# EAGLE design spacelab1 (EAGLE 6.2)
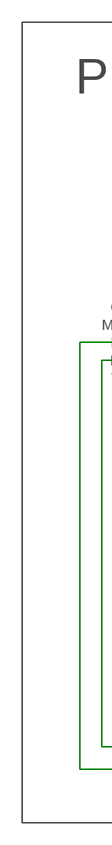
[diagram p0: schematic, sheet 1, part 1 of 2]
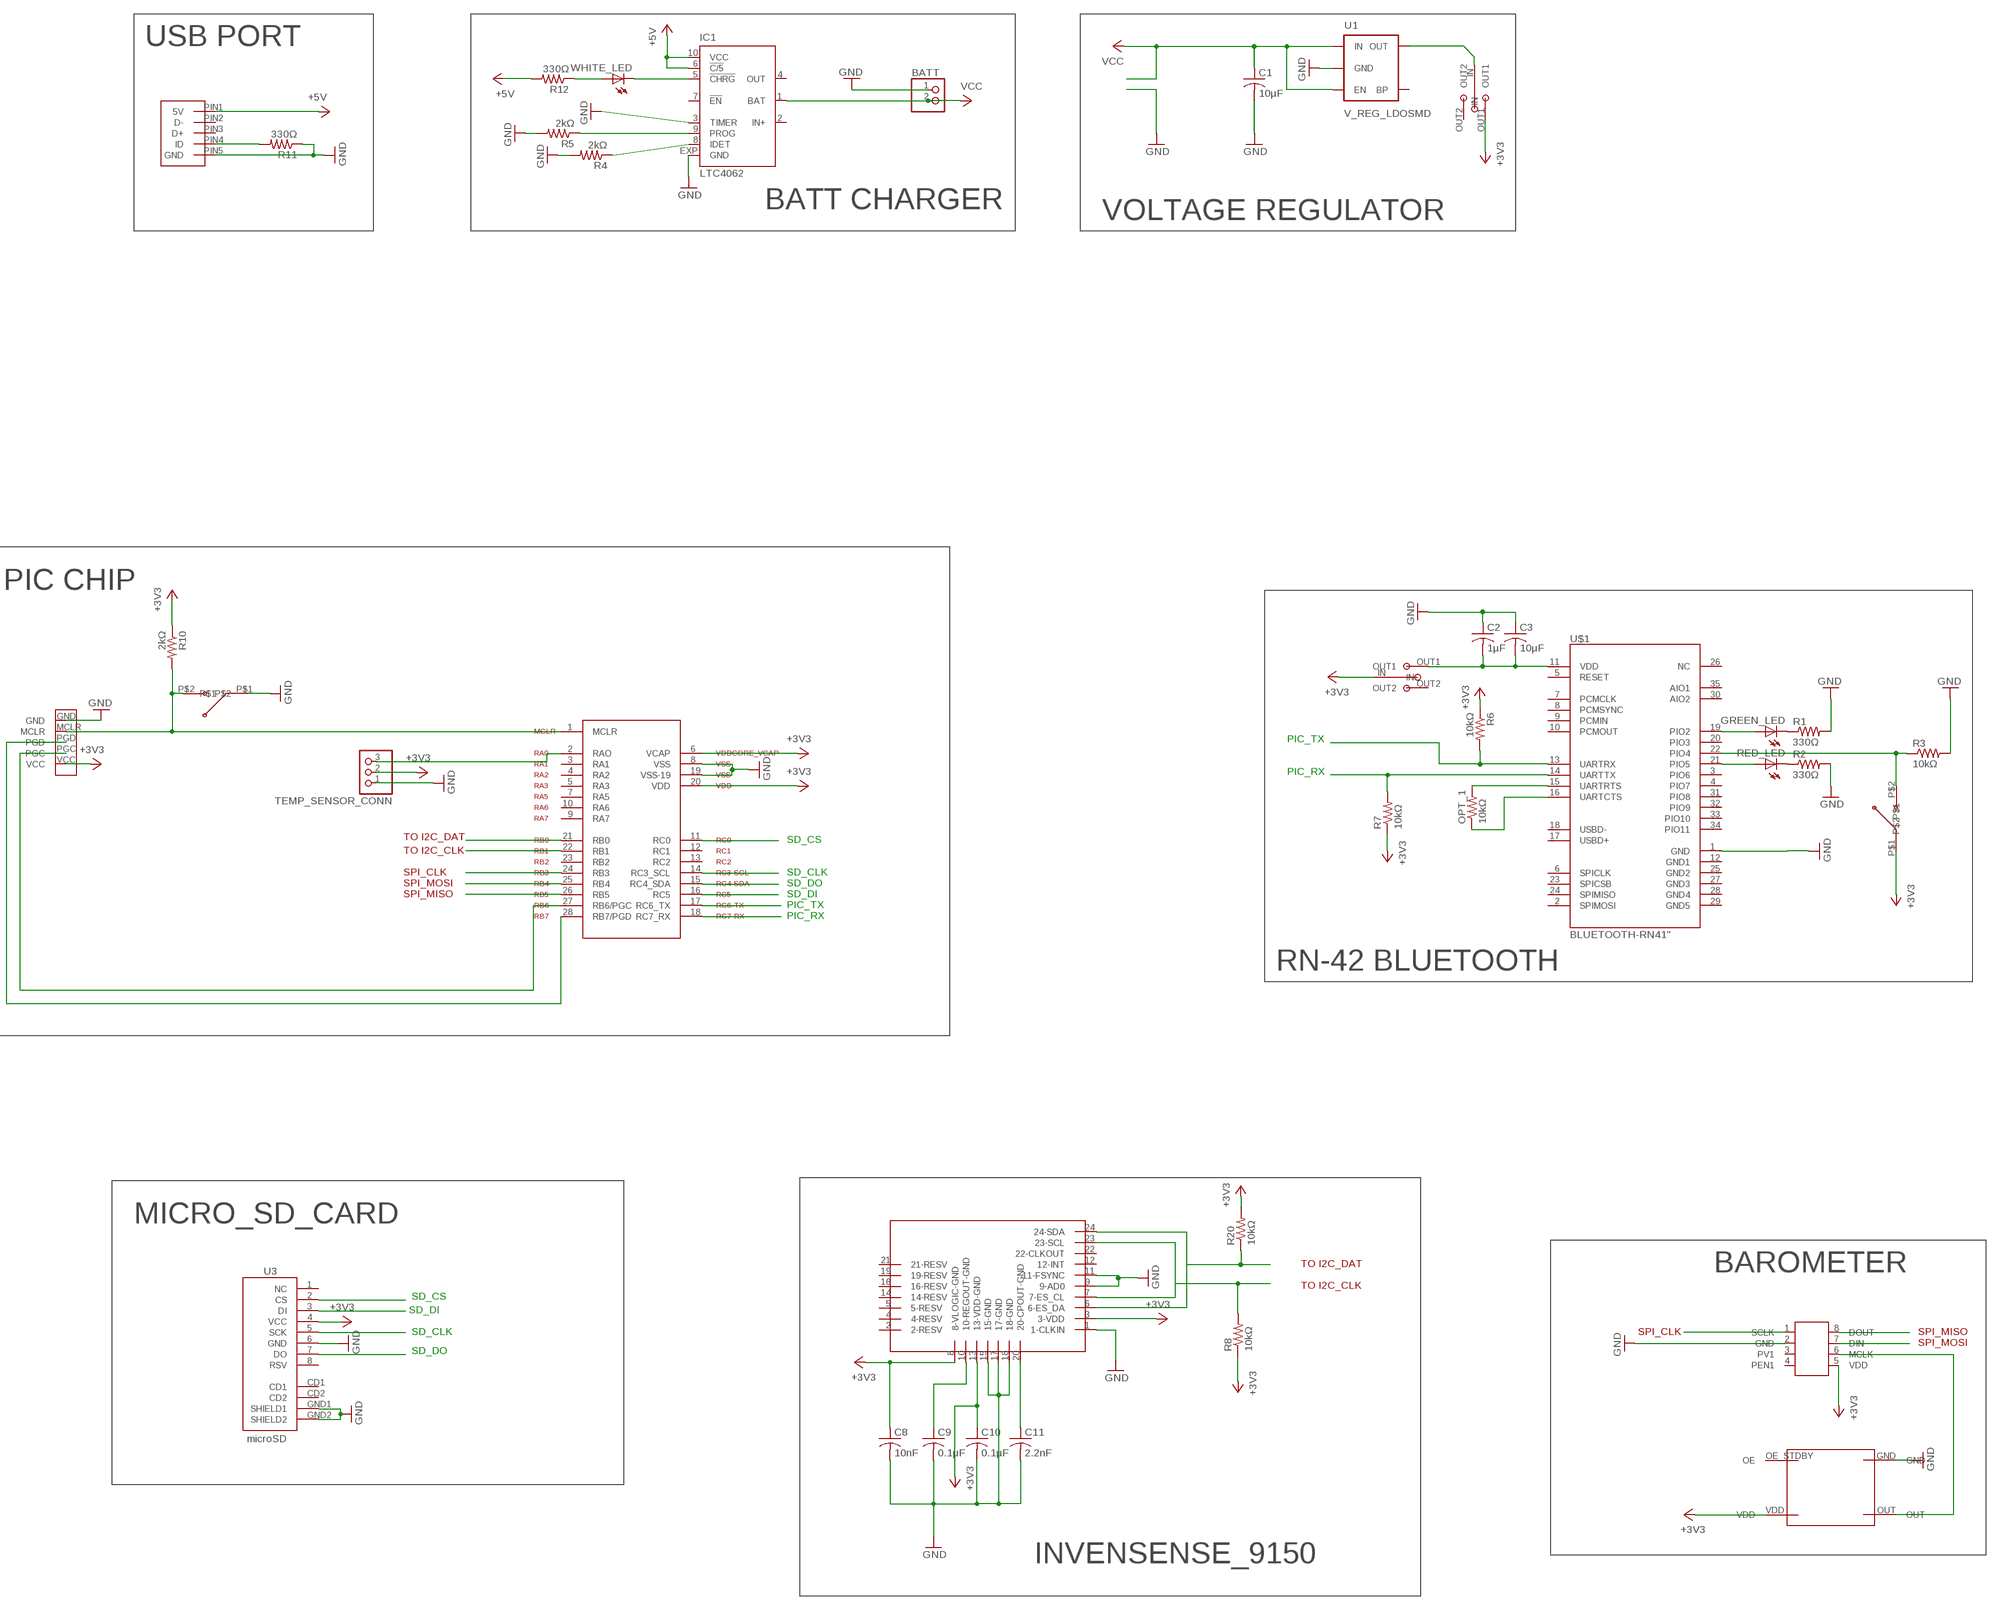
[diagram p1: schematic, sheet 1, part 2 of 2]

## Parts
BATT  PINHD-1X2  [1X02]
BT_PWR  CUS12TB_LOW_PROFILE_SWITCH  [CUS12TB_FOOTPRINT]
BT_RST  KSR211_MOM  [KSR_211_FOOTPRINT]
C1  10µF  C-USC0603  [C0603]
C2  1µF  C-USC0603  [C0603]
C3  10µF  C-USC0603  [C0603]
C8  10nF  C-USC0805  [C0805]
C9  0.1µF  C-USC0805  [C0805]
C10  0.1µF  C-USC0805  [C0805]
C11  2.2nF  C-USC0805  [C0805]
GREEN_LED  LEDCHIP-LED0805  [CHIP-LED0805]
IC1  LTC4062  [DFN10-3X3]
MAIN_PWR  CUS12TB_LOW_PROFILE_SWITCH  [CUS12TB_FOOTPRINT]
OPT_1  10kΩ  R-US_R0603  [R0603]
PIC18F26J11  PIC18F26J11  [SSOP-28]
PIC_RST  KSR211_MOM  [KSR_211_FOOTPRINT]
R1  330Ω  R-US_R0603  [R0603]
R2  330Ω  R-US_R0603  [R0603]
R3  10kΩ  R-US_R0603  [R0603]
R4  2kΩ  R-US_R0603  [R0603]
R5  2kΩ  R-US_R0603  [R0603]
R6  10kΩ  R-US_R0603  [R0603]
R7  10kΩ  R-US_R0603  [R0603]
R8  10kΩ  R-US_R0603  [R0603]
R10  2kΩ  R-US_R0603  [R0603]
R11  330Ω  R-US_R0603  [R0603]
R12  330Ω  R-US_R0603  [R0603]
R20  10kΩ  R-US_R0603  [R0603]
RED_LED  LEDCHIP-LED0805  [CHIP-LED0805]
TEMP_SENSOR_CONN  PINHD-1X3  [1X03]
U1  V_REG_LDOSMD  [SOT23-5]
U3  microSD  USD-SOCKETSMD  [MICRO-SD-SOCKET-PP]
U$1  BLUETOOTH-RN41"  [RN41]
U$2  CSX_750F_CLOCK  [CITIZEN_CSX-750_CRYSTAL_OSCILLATOR]
U$3  5-PAD_PROG_HEAD  [5-BUTTON_PAD]
U$4  INVENSENSE-MPU9150  [INVENSENSE-MPU9150]
U$5  WURTH_MICRO_USB_SMD  [MICRO_USB_SMD]
U$8  MS5540C_BAROMETER  [8_PIN_MS5540C]
WHITE_LED  LEDCHIP-LED0805  [CHIP-LED0805]

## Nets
+3V3: BT_PWR.IN BT_RST.P$1 C8.1 C10.1 MAIN_PWR.OUT1 PIC18F26J11.6(VCAP) PIC18F26J11.20(VDD) R6.1 R7.1 R8.1 R10.1 R20.2 TEMP_SENSOR_CONN.2 U3.4(VCC) U$2.VDD U$3.VCC U$4.3(3-VDD) U$4.8(8-VLOGIC-GND) U$4.13(13-VDD-GND) U$8.5(VDD)
+5V: IC1.6(!C/5) IC1.10(VCC) R12.2 U$5.PIN1(5V)
GND: BATT.1 C1.2 C2.1 C3.1 C8.2 C9.2 C10.2 C11.2 IC1.3(TIMER) IC1.EXP(GND) PIC18F26J11.8(VSS) PIC18F26J11.19(VSS-19) PIC_RST.P$1 R1.2 R2.2 R3.2 R4.2 R5.2 R11.1 TEMP_SENSOR_CONN.1 U1.2(GND) U3.6(GND) U3.GND1(SHIELD1) U3.GND2(SHIELD2) U$1.1(GND) U$2.GND U$3.GND U$4.1(1-CLKIN) U$4.9(9-AD0) U$4.11(11-FSYNC) U$4.15(15-GND) U$4.17(17-GND) U$4.18(18-GND) U$5.PIN5(GND) U$8.2(GND)
I2C_CLK: PIC18F26J11.22(RB1) R8.2 U$4.7(7-ES_CL) U$4.23(23-SCL)
I2C_DAT: PIC18F26J11.21(RB0) R20.1 U$4.6(6-ES_DA) U$4.24(24-SDA)
N$1: GREEN_LED.A U$1.19(PIO2)
N$2: RED_LED.A U$1.21(PIO5)
N$3: GREEN_LED.C R1.1
N$4: R2.1 RED_LED.C
N$5: BT_RST.P$2 R3.1 U$1.22(PIO4)
N$6: OPT_1.2 U$1.15(UARTRTS)
N$7: OPT_1.1 U$1.16(UARTCTS)
N$8: IC1.9(PROG) R5.1
N$9: IC1.8(IDET) R4.1
N$10: U$8.1(SCLK)
N$11: R11.2 U$5.PIN4(ID)
N$12: U$8.7(DIN)
N$13: PIC18F26J11.1(MCLR) PIC_RST.P$2 R10.2 U$3.MCLR
N$14: U$8.8(DOUT)
N$15: PIC18F26J11.28(RB7/PGD) U$3.PGD
N$16: PIC18F26J11.27(RB6/PGC) U$3.PGC
N$17: PIC18F26J11.2(RAO) TEMP_SENSOR_CONN.3
N$18: BT_PWR.OUT1 C2.2 C3.2 U$1.11(VDD)
N$19: U$2.OUT U$8.6(MCLK)
N$23: IC1.5(!CHRG) WHITE_LED.C
N$24: R12.1 WHITE_LED.A
N$29: MAIN_PWR.IN U1.5(OUT)
N$44: C9.1 U$4.10(10-REGOUT-GND)
N$45: C11.1 U$4.20(20-CPOUT-GND)
PIC_RX: PIC18F26J11.18(RC7_RX) R7.2 U$1.14(UARTTX)
PIC_TX: PIC18F26J11.17(RC6_TX) R6.2 U$1.13(UARTRX)
SD_CLK: PIC18F26J11.14(RC3_SCL) U3.5(SCK)
SD_CS: PIC18F26J11.11(RC0) U3.2(CS)
SD_DI: PIC18F26J11.16(RC5) U3.3(DI)
SD_DO: PIC18F26J11.15(RC4_SDA) U3.7(DO)
SPI_CLK: PIC18F26J11.24(RB3)
SPI_MISO: PIC18F26J11.26(RB5)
SPI_MOSI: PIC18F26J11.25(RB4)
VCC: BATT.2 C1.1 IC1.1(BAT) U1.1(IN) U1.3(EN)
Unconnected: BT_PWR.OUT2 IC1.2(IN+) IC1.4(OUT) IC1.7(!EN) MAIN_PWR.OUT2 PIC18F26J11.3(RA1) PIC18F26J11.4(RA2) PIC18F26J11.5(RA3) PIC18F26J11.7(RA5) PIC18F26J11.9(RA7) PIC18F26J11.10(RA6) PIC18F26J11.12(RC1) PIC18F26J11.13(RC2) PIC18F26J11.23(RB2) U1.4(BP) U3.1(NC) U3.8(RSV) U3.CD1 U3.CD2 U$1.2(SPIMOSI) U$1.3(PIO6) U$1.4(PIO7) U$1.5(RESET) U$1.6(SPICLK) U$1.7(PCMCLK) U$1.8(PCMSYNC) U$1.9(PCMIN) U$1.10(PCMOUT) U$1.12(GND1) U$1.17(USBD+) U$1.18(USBD-) U$1.20(PIO3) U$1.23(SPICSB) U$1.24(SPIMISO) U$1.25(GND2) U$1.26(NC) U$1.27(GND3) U$1.28(GND4) U$1.29(GND5) U$1.30(AIO2) U$1.31(PIO8) U$1.32(PIO9) U$1.33(PIO10) U$1.34(PIO11) U$1.35(AIO1) U$2.OE_STDBY(OE) U$4.2(2-RESV) U$4.4(4-RESV) U$4.5(5-RESV) U$4.12(12-INT) U$4.14(14-RESV) U$4.16(16-RESV) U$4.19(19-RESV) U$4.21(21-RESV) U$4.22(22-CLKOUT) U$5.PIN2(D-) U$5.PIN3(D+) U$8.3(PV1) U$8.4(PEN1)

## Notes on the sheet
- USB PORT
- BATT CHARGER
- VOLTAGE REGULATOR
- PIC CHIP
- PIC_TX
- PIC_RX
- TO I2C_DAT | SD_CS
- TO I2C_CLK
- SPI_CLK | SD_CLK
- SPI_MOSI | SD_DO
- SPI_MISO | SD_DI
- PIC_TX
- PIC_RX
- RN-42 BLUETOOTH
- MICRO_SD_CARD
- TO I2C_DAT
- BAROMETER
- TO I2C_CLK
- SD_CS
- SD_DI
- SD_CLK | SPI_CLK | SPI_MISO
- SPI_MOSI
- SD_DO
- INVENSENSE_9150

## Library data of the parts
BATT = pinhead:PINHD-1X2: PIN HEADER
BT_PWR MAIN_PWR = copal_slide_switches:CUS12TB_LOW_PROFILE_SWITCH
BT_RST PIC_RST = c_and_k_switches:KSR211_MOM
C1-C3 C8-C11 = resistor:C-US: CAPACITOR, American symbol
GREEN_LED RED_LED WHITE_LED = led:LED: LED
IC1 = linear-technology:LTC4062: Standalone Linear Li-Ion Battery Charger with Micropower Comparator Source: http://www.linear.com .. 4062fa.pdf; MPN: LTC4062EDD#PBF; OC_FARNELL: 1648037; OC_NEWARK: 58M0900
OPT_1 R1-R8 R10-R12 R20 = resistor:R-US_: RESISTOR, American symbol
PIC18F26J11 = 18F26J11:PIC18F26J11
TEMP_SENSOR_CONN = pinhead:PINHD-1X3: PIN HEADER
U1 = SparkFun-PowerIC:V_REG_LDO: Voltage Regulator LDO Standard 150mA LDO voltage regulator in SOT-23 layout. Micrel part MIC5205. BP (by-pass) pin is used to lower output noise with 470pF cap.
U3 = SparkFun:USD-SOCKET: microSD Socket Push-push type uSD socket. Schematic element and footprint production proven. Spark Fun Electronics SKU : PRT-00127. tDoc lines correctly indicate media card edge positions when inserting (unlocked, locked, depressed).
U$1 = SparkFun-RF:BLUETOOTH-RN41: Bluetooth SMD module
U$2 = citizen:CSX_750F_CLOCK
U$3 = Jeremy_Parts:5-PAD_PROG_HEAD
U$4 = vids-parts:INVENSENSE-MPU9150
U$5 = wurth_micro_usb:WURTH_MICRO_USB_SMD
U$8 = Intersema:MS5540C_BAROMETER

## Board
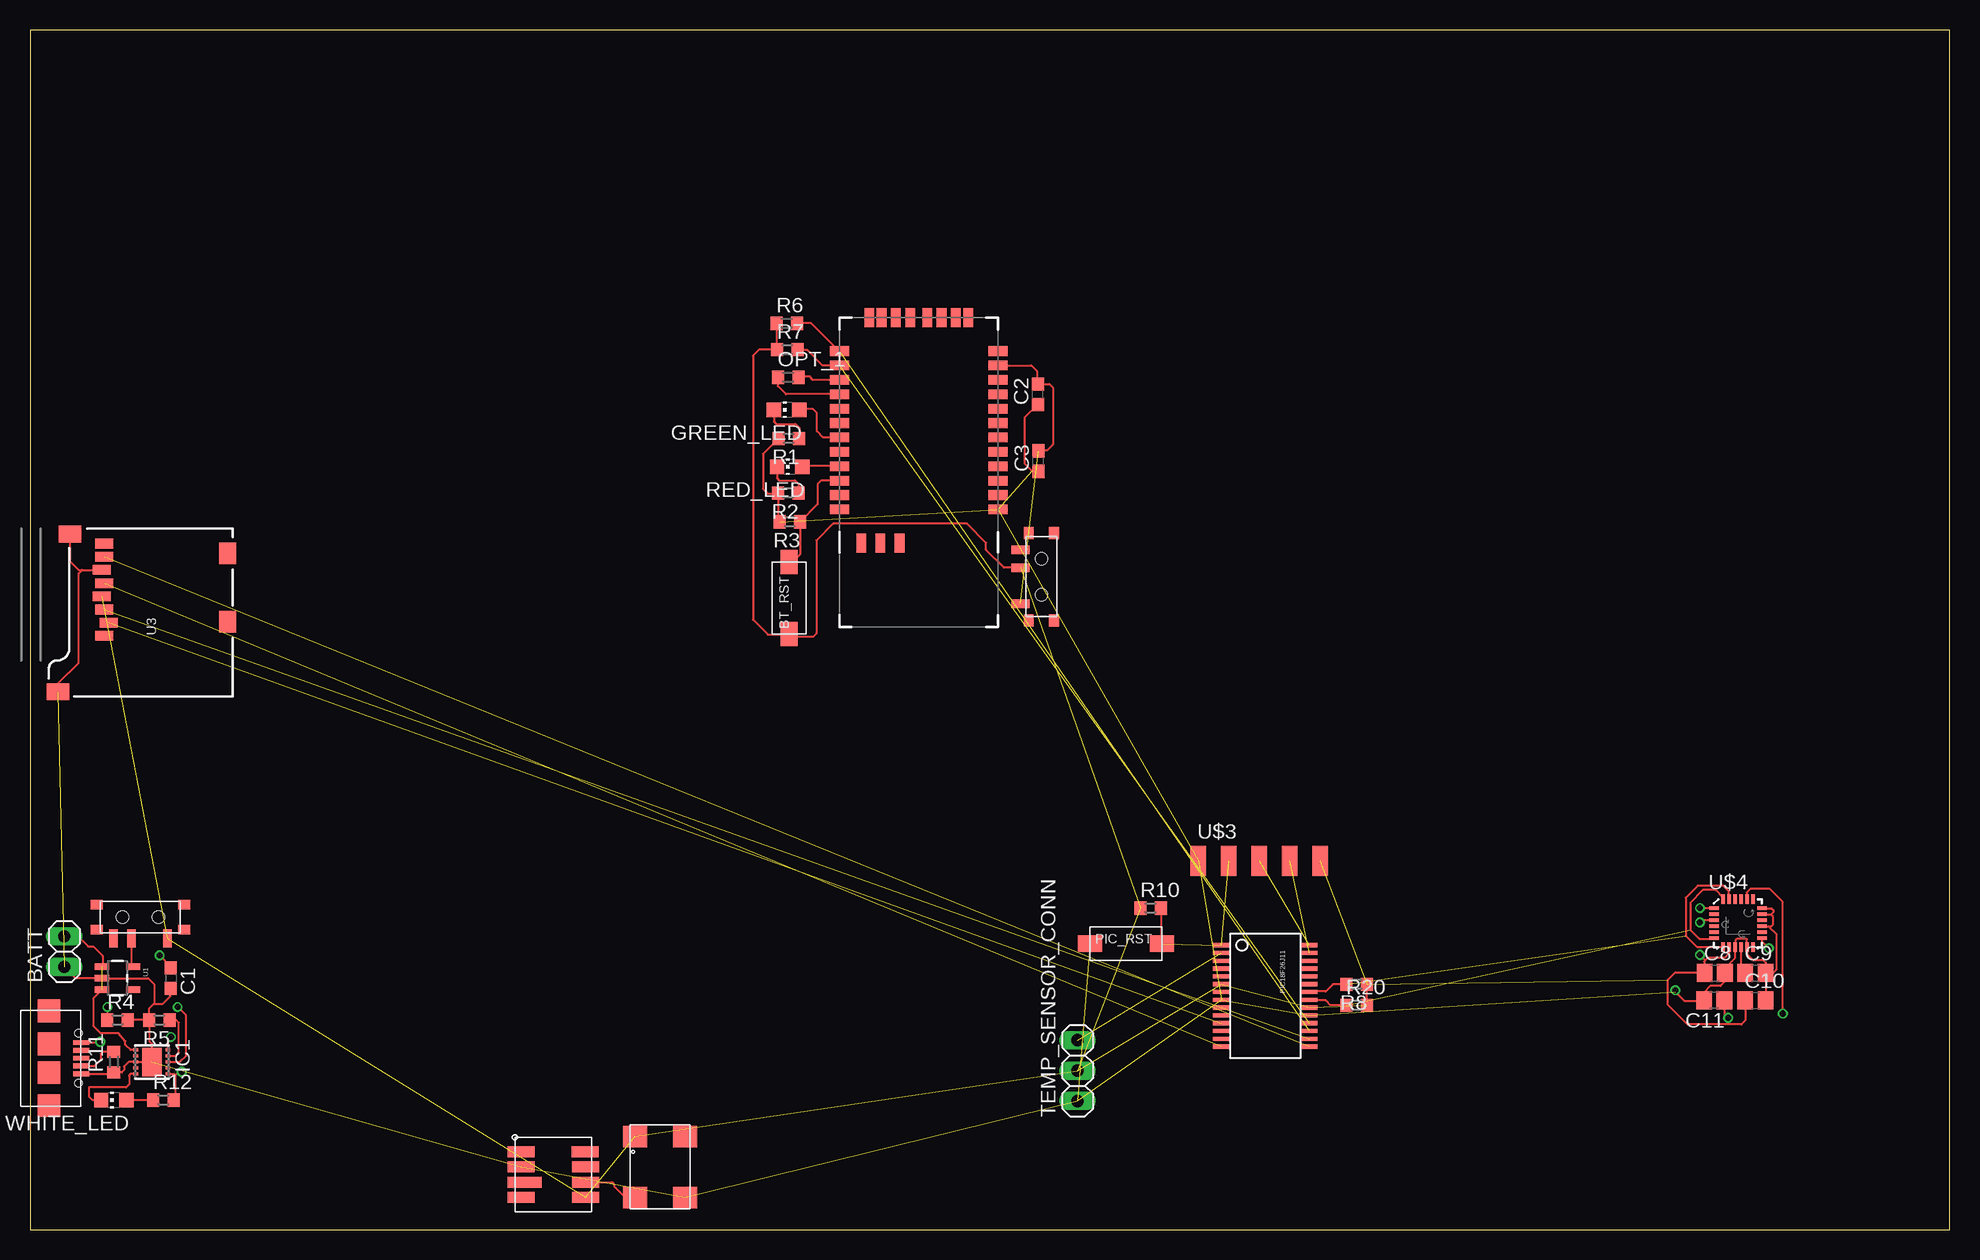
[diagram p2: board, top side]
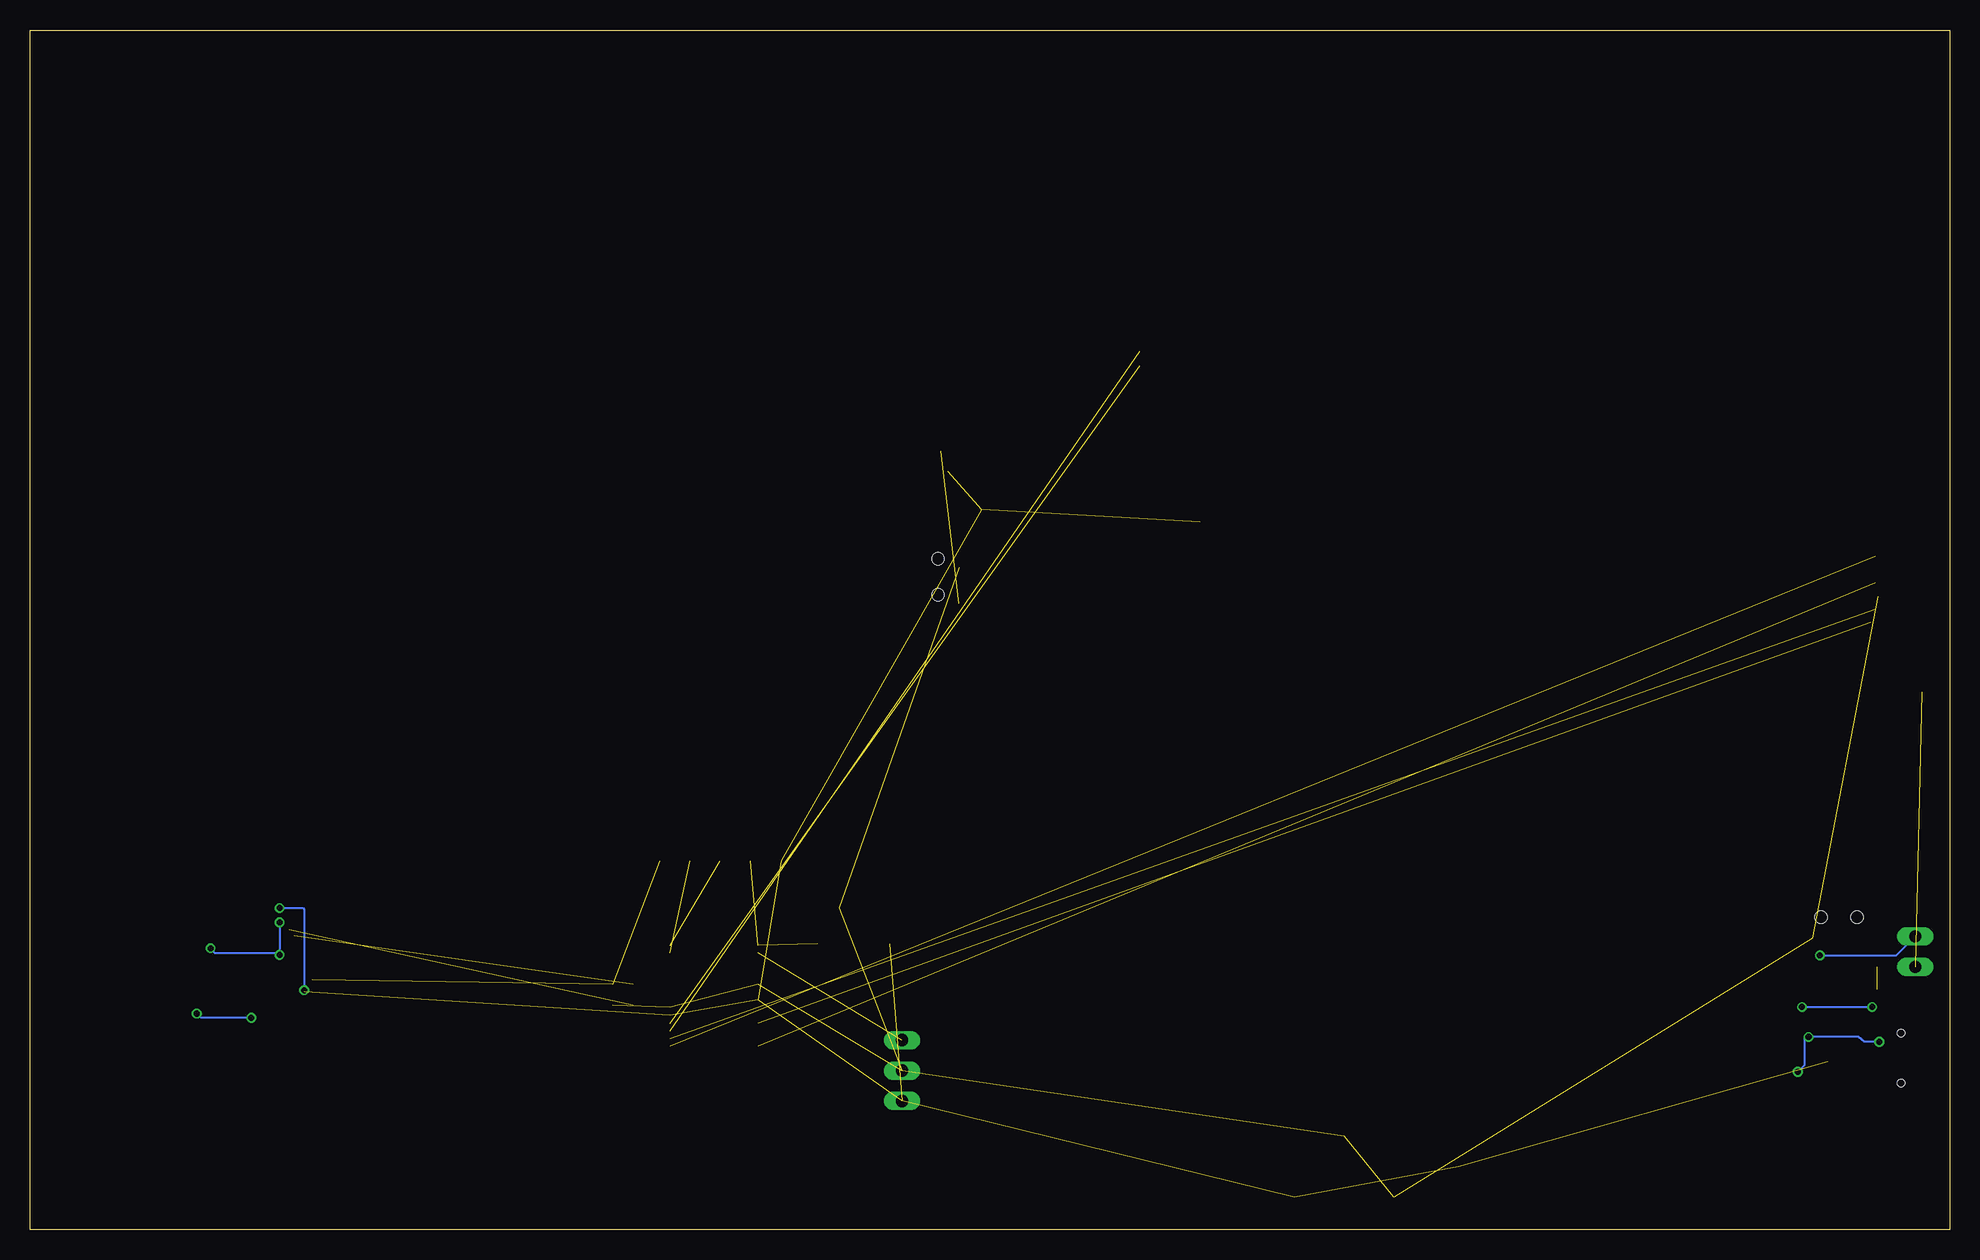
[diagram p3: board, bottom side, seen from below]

Size 160 x 100 mm. Coordinates in mm from the lower left corner, seen from the top.
Outline: 0,0 160,0 160,100 0,100 0,0
Copper layers (1*16): Top 0.035mm / dielectric 1.5mm / Bottom 0.035mm
Design rules: minimum track width 6mil, minimum drill 12mil, track to track 6mil, track to pad 6mil, pad to pad 6mil, via to via 6mil, smd to smd 6mil, copper to edge 10mil, drill to drill 10mil, minimum pad ring 10mil, minimum via ring 6mil, stop-mask expansion 2mil, vias tented up to drill 100mil, thermal gap 10mil

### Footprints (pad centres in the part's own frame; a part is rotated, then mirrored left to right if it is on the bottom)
1X02 = drill 1.016 long: 1 -1.27,0; 2 1.27,0
CUS12TB_FOOTPRINT = smd 0.7 x 1.5: IN 0.75,1.75; OUT1 -2.25,1.75; OUT2 2.25,1.75 | smd 1 x 0.8: NC1 -3.65,1.05; NC2 -3.65,-1.05; NC3 3.65,1.05; NC4 3.65,-1.05 | hole 1: -1.5,0; 1.5,0
KSR_211_FOOTPRINT = smd 2 x 1.4: P$1 -3,0; P$2 3,0
C0603 = smd 1.1 x 1: 1 -0.85,0; 2 0.85,0
C0805 = smd 1.3 x 1.5: 1 -0.85,0; 2 0.85,0
CHIP-LED0805 = smd 1.2 x 1.2: A 0,-1.05; C 0,1.05
DFN10-3X3 = smd 0.25 x 0.45: 1 -1,-1.35; 2 -0.5,-1.35; 3 0,-1.35; 4 0.5,-1.35; 5 1,-1.35; 6 1,1.35; 7 0.5,1.35; 8 0,1.35; 9 -0.5,1.35; 10 -1,1.35 | smd 2.38 x 1.65: EXP 0,0
R0603 = smd 1 x 1.1: 1 -0.85,0; 2 0.85,0
SSOP-28 = smd 0.348 x 1.397: 1 -4.225,-3.656; 2 -3.575,-3.656; 3 -2.925,-3.656; 4 -2.275,-3.656; 5 -1.625,-3.656; 6 -0.975,-3.656; 7 -0.325,-3.656; 8 0.325,-3.656; 9 0.975,-3.656; 10 1.625,-3.656; 11 2.275,-3.656; 12 2.925,-3.656; 13 3.575,-3.656; 14 4.225,-3.656; 15 4.225,3.656; 16 3.575,3.656; 17 2.925,3.656; 18 2.275,3.656; 19 1.625,3.656; 20 0.975,3.656; 21 0.325,3.656; 22 -0.325,3.656; 23 -0.975,3.656; 24 -1.625,3.656; 25 -2.275,3.656; 26 -2.925,3.656; 27 -3.575,3.656; 28 -4.225,3.656
1X03 = drill 1.016 long: 1 -2.54,0; 2 0,0; 3 2.54,0
SOT23-5 = smd 0.55 x 1.2: 1 -0.95,-1.3; 2 0,-1.3; 3 0.95,-1.3; 4 0.95,1.3; 5 -0.95,1.3
MICRO-SD-SOCKET-PP = smd 0.8 x 1.5: 1 -8.94,10.7; 2 -7.84,10.3; 3 -6.74,10.7; 4 -5.64,10.9; 5 -4.54,10.7; 6 -3.44,10.9; 7 -2.34,10.7; 8 -1.24,10.7 | smd 1.8 x 1.4: CD1 -7.75,0.4; CD2 -2.05,0.4 | smd 1.4 x 1.9: GND1 -13.6,14.55; GND2 -0.45,13.55
RN41 = smd 0.8 x 1.6: 1 -6.6,-6.6; 2 -5.4,-6.6; 3 -4.2,-6.6; 4 -3,-6.6; 5 -1.8,-6.6; 6 -0.6,-6.6; 7 0.6,-6.6; 8 1.8,-6.6; 9 3,-6.6; 10 4.2,-6.6; 11 5.4,-6.6; 12 6.6,-6.6; 13 6.6,6.6; 14 5.4,6.6; 15 4.2,6.6; 16 3,6.6; 17 1.8,6.6; 18 0.6,6.6; 19 -0.6,6.6; 20 -1.8,6.6; 21 -3,6.6; 22 -4.2,6.6; 23 -5.4,6.6; 24 -6.6,6.6 | smd 1.6 x 0.8: 25 -9.4,4.8; 26 -9.4,3.2; 27 -9.4,1.6; 28 9.4,3.1; 29 9.4,-3.1; 30 9.4,-4.122; 31 9.4,-1.9; 32 9.4,-0.7; 33 9.4,0.7; 34 9.4,1.9; 35 9.4,4.122
CITIZEN_CSX-750_CRYSTAL_OSCILLATOR = smd 1.8 x 2: GND 2.54,2.1; OE_STDBY -2.54,2.1; OUT 2.54,-2.1; VDD -2.54,-2.1
5-BUTTON_PAD = smd 1.27 x 2.54: GND -6.35,0; MCLR -3.81,0; PGC 1.27,0; PGD -1.27,0; VCC 3.81,0
INVENSENSE-MPU9150 = smd 0.8 x 0.3: 1 -2,1.25; 2 -2,0.75; 3 -2,0.25; 4 -2,-0.25; 5 -2,-0.75; 6 -2,-1.25; 13 2,-1.25; 14 2,-0.75; 15 2,-0.25; 16 2,0.25; 17 2,0.75; 18 2,1.25 | smd 0.3 x 0.8: 7 -1.25,-2; 8 -0.75,-2; 9 -0.25,-2; 10 0.25,-2; 11 0.75,-2; 12 1.25,-2; 19 1.25,2; 20 0.75,2; 21 0.25,2; 22 -0.25,2; 23 -0.75,2; 24 -1.25,2
MICRO_USB_SMD = smd 1.9 x 1.9: NC1 -3.95,0; NC2 -1.2,0; NC3 1.2,0; NC4 3.95,0 | smd 0.4 x 1.35: PIN1 -1.3,2.675; PIN2 -0.65,2.675; PIN3 0,2.675; PIN4 0.65,2.675; PIN5 1.3,2.675 | hole 0.6: -2.075,2.45; 2.075,2.45
8_PIN_MS5540C = smd 2.25 x 0.9: 1 -2.675,0; 2 -2.675,-1.25; 4 -2.675,-3.8; 5 2.675,-3.8; 6 2.675,-2.55; 7 2.675,-1.25; 8 2.625,0 | smd 2.8 x 0.9: 3 -2.4,-2.55

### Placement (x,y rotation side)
BATT  2.86,23.18 90 top
BT_PWR  84.31,54.42 90 top
BT_RST  63.27,52.63 90 top
C1  11.75,20.95 270 top
C2  84,69.63 90 top
C3  84.05,64.06 90 top
C8  140.42,21.4 0 top
C9  143.82,21.4 0 top
C10  143.82,19.1 0 top
C11  140.38,19.1 180 top
GREEN_LED  63.06,68.35 90 top
IC1  10.16,13.97 270 top
MAIN_PWR  9.21,26.04 180 top
OPT_1  63.2,71.05 0 top
PIC18F26J11  102.97,19.48 270 top
PIC_RST  91.34,23.83 0 top
R1  63.25,65.95 180 top
R2  63.2,61.4 180 top
R3  63.33,59 180 top
R4  7.3,17.46 0 top
R5  10.79,17.46 180 top
R6  63.07,75.55 0 top
R7  63.12,73.35 0 top
R8  110.58,20.45 180 top
R10  93.41,26.8 0 top
R11  6.99,13.97 90 top
R12  11.11,10.79 0 top
R20  110.57,18.7 0 top
RED_LED  63.32,63.6 90 top
TEMP_SENSOR_CONN  87.32,13.25 90 top
U1  7.3,20.95 270 top
U3  16.88,58.43 90 top
U$1  74.08,66.63 90 top
U$2  52.52,5.22 270 top
U$3  103.73,30.73 0 top
U$4  142.36,25.54 0 top
U$5  1.59,14.29 270 top
U$8  43.63,6.49 0 top
WHITE_LED  6.99,10.79 90 top

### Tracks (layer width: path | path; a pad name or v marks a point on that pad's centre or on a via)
+3V3  (via drill 0.51)  (11 unrouted)
  Top 0.152: R20.2 R8.1 | U$4.8 141.61,23.01 141.25,22.65 139.85,22.65 139.62,22.43 | 139.62,22.43 139.55,22.35 139.55,21.42 C8.1 139.52,21.45 137.15,21.45 136.5,20.8 136.5,18.75 138.15,17.1 142.65,17.1 142.97,17.42 C10.1 | U$4.3 139.39,25.79 v139.2,25.6 | v139.2,22.9 139.2,22.85 139.62,22.43 | U$4.13 144.36,24.04 v144.95,23.45 | R6.1 62.22,73.4 R7.1 60.75,73.35 60.25,72.85 60.25,50.85 61.5,49.6 63.24,49.6 BT_RST.P$1 63.5,49.4 65.25,49.4 65.55,49.7 65.55,57.45 66.95,58.85 78.1,58.85 79.7,57.25 79.7,56.65 81.18,55.17 BT_PWR.IN
  Bottom 0.152: v139.2,25.6 v139.2,22.9 139.35,23.05 144.6,23.05 144.95,23.4 v144.95,23.45
+5V  (via drill 0.51)
  Top 0.152: IC1.6 11.98,12.97 12.1,12.85 | 12.1,12.85 12.1,10.93 R12.2 | IC1.10 11.51,15.81 v11.75,16.05 | v12.65,13.15 12.4,13.15 12.1,12.85 | U$5.PIN1 5.61,15.59 v5.85,15.65
  Bottom 0.152: v12.65,13.15 12.1,13.7 12.1,15.9 11.95,16.05 v11.75,16.05 7.6,16.05 7.1,15.65 v5.85,15.65
GND  (via drill 0.51)  (12 unrouted)
  Top 0.152: U$5.PIN5 6.85,12.99 R11.1 7,13.1 7.65,13.1 7.85,13.3 7.85,13.6 8.22,13.97 IC1.3 IC1.EXP 10.15,15.5 9.95,15.71 R5.2 | R5.2 9.95,18.45 10.3,18.8 | 10.3,18.8 11.05,18.8 11.7,19.45 11.7,20.06 C1.2 | R5.2 R4.2 | BATT.1 3.81,20.95 U1.2 9.85,20.95 10.35,20.45 10.35,18.85 10.3,18.8 | U3.GND2 3.33,55.72 4.05,55 4.35,55 | 4.35,55 U3.6 | U3.GND1 2.33,45.53 4.05,47.25 4.05,54.7 4.35,55 | U$4.18 145.16,26.79 145.3,26.65 145.3,26.45 145.1,26.25 | 145.1,26.25 144.4,26.25 U$4.17 | 145.1,26.25 145.3,26.05 145.3,25.45 145.14,25.29 U$4.15 144.91,25.29 145.55,24.65 145.55,21.65 145.3,21.4 C9.2 | C9.2 144.7,21.43 144.7,22.25 144.45,22.5 143.6,22.5 143.11,22.99 U$4.11 143.11,24.19 143.05,24.25 142.3,24.25 142.15,24.1 142.15,23.58 U$4.9 142.11,22.61 141.7,22.2 141.7,21.83 C8.2 141.27,20.67 140.9,20.3 140.05,20.3 139.5,19.75 139.5,19.13 C11.2 139.48,19.05 137.9,19.05 137.15,19.8 v137.15,19.95 | C9.2 C10.2 | U$4.1 v139.21,26.79 v139.2,26.8 | C3.1 83.54,63.21 82.95,63.8 82.95,67.73 C2.1 | R3.2 62.35,59.13 R2.2 62.3,61.35 61.5,61.35 61.1,61.75 61.1,64.65 R1.2
  Bottom 0.152: v139.2,26.8 137.25,26.8 137.15,26.7 v137.15,19.95
I2C_CLK  (1 unrouted)
  Top 0.152: R8.2 108.6,20.45 108,19.85 106.67,19.85 PIC18F26J11.22 | U$4.23 141.61,28.19 141.15,28.65 139,28.65 138,27.65 138,24.5 138.95,23.55 U$4.7
I2C_DAT  (1 unrouted)
  Top 0.152: R20.1 108.4,18.7 108,19.1 106.68,19.1 PIC18F26J11.21 | U$4.24 141.11,27.69 140.5,28.3 139.45,28.3 138.4,27.25 138.4,25 139.15,24.25 140.32,24.25 U$4.6
N$1
  Top 0.152: U$1.19 66.12,66.03 65.6,66.55 65.6,68.05 65.25,68.4 64.16,68.4 GREEN_LED.A
N$2
  Top 0.152: U$1.21 64.4,63.63 RED_LED.A
N$3
  Top 0.152: GREEN_LED.C 62.01,67.34 62.2,67.15 63.8,67.15 64.15,66.8 64.15,66 R1.1
N$4
  Top 0.152: RED_LED.C 62.27,62.63 62.45,62.45 63.75,62.45 64.05,62.15 R2.1
N$5
  Top 0.152: U$1.22 65.93,62.43 65.65,62.15 65.65,60.47 R3.1 64.18,56.28 63.8,55.9 63.54,55.9 BT_RST.P$2
N$6
  Top 0.152: U$1.15 65.27,70.83 65,71.1 64.1,71.1 OPT_1.2
N$7
  Top 0.152: U$1.16 63.02,69.63 62.35,70.3 OPT_1.1
N$8
  Top 0.152: IC1.9 12.12,14.47 12.4,14.75 12.4,17.25 12.2,17.45 11.66,17.45 R5.1
N$9  (via drill 0.51)
  Top 0.152: IC1.8 12.47,13.97 13,14.5 13,17.85 v12.3,18.55 | v6.45,18.55 R4.1
  Bottom 0.152: v12.3,18.55 v6.45,18.55
N$11
  Top 0.152: R11.2 6.07,14.82 5.9,14.65 5.9,14.15 5.35,13.6 4.3,13.6 U$5.PIN4
N$13  (2 unrouted)
  Top 0.152: R10.2 94.26,23.91 PIC_RST.P$2
N$15  (1 unrouted)
N$16  (1 unrouted)
N$17  (1 unrouted)
N$18  (1 unrouted)
  Top 0.152: U$1.11 83.47,72.03 83.95,71.55 83.95,70.53 C2.2 84.97,70.48 85.25,70.2 85.25,65.45 84.75,64.95 84.09,64.95 C3.2
N$19
  Top 0.152: U$8.6 48.51,3.94 48.7,3.75 48.7,3.6 49.6,2.7 50.4,2.7 U$2.OUT
N$23
  Top 0.152: IC1.5 8.37,12.97 8.25,12.85 8.25,12.1 8,11.85 4.95,11.85 4.9,11.8 4.9,11.1 5.2,10.8 WHITE_LED.C
N$24
  Top 0.152: WHITE_LED.A R12.1
N$29
  Top 0.152: MAIN_PWR.IN 8.46,22.05 U1.5
N$44
  Top 0.152: U$4.10 142.61,21.76 C9.1
N$45  (via drill 0.51)
  Top 0.152: C11.1 141.23,17.97 v141.55,17.65 | v146.1,18 146.1,27.3 145,28.4 143.4,28.4 143.1,28.1 U$4.20
  Bottom 0.152: v141.55,17.65 145.75,17.65 v146.1,18
PIC_RX  (1 unrouted)
  Top 0.152: U$1.14 66.07,72.03 64.8,73.3 64.02,73.3 R7.2
PIC_TX  (1 unrouted)
  Top 0.152: U$1.13 67.42,73.23 65.1,75.55 R6.2
SD_CLK  (1 unrouted)
SD_CS  (1 unrouted)
SD_DI  (1 unrouted)
SD_DO  (1 unrouted)
VCC  (via drill 0.51)  (1 unrouted)
  Top 0.152: BATT.2 4,24.45 4.85,23.6 5.25,23.6 6.05,22.8 6.05,21.95 U1.1 | C1.1 11.75,21.9 v10.8,22.85 | IC1.1 8.38,14.97 7.95,15.4 7.95,15.7 7.4,16.35 5.9,16.35 5.3,16.95 5.3,19.3 U1.3
  Bottom 0.152: v10.8,22.85 4.46,22.85 BATT.2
